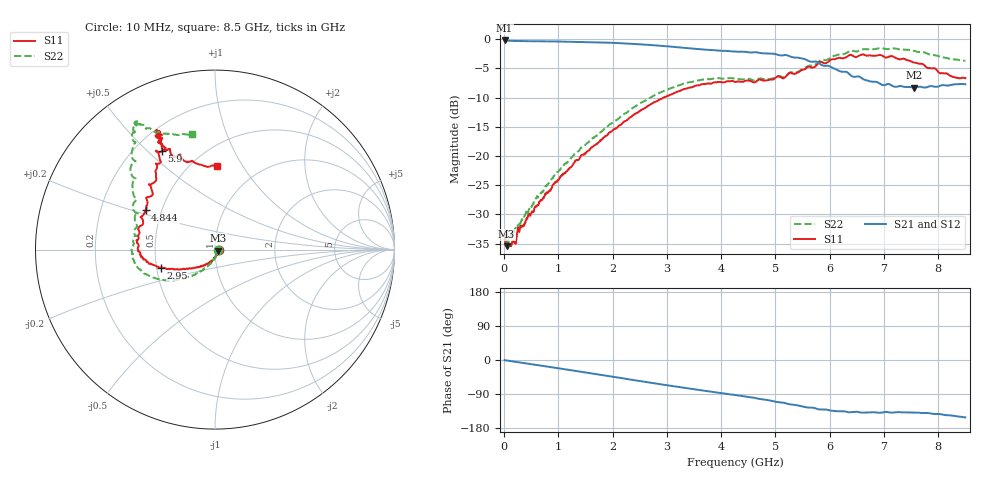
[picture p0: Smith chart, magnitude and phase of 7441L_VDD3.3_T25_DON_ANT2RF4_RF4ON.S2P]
!Agilent Technologies,E5071C,MY46417908,A.11.23
!Date: Mon May 03 19:54:53 2021
!Data & Calibration Information:
!Freq	S11:SOLT2(ON)	S21:SOLT2(ON)	S12:SOLT2(ON)	S22:SOLT2(ON)
!PortZ  Port1:50+j0  Port2:50+j0
!Above PortZ is port z conversion or system Z0 setting when saving the data.
!When reading, reference impedance value at option line is always used.
# Hz S dB R 50
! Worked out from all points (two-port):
!   1601 points, 10 MHz to 8.5 GHz, reference 50 ohm
!   highest |S21| = -0.21 dB at 10 MHz (marker M1); lowest = -8.3 dB at 7.561 GHz (marker M2)
!   |S21| within 3 dB of the highest: start of sweep to 5.456 GHz
!   lowest |S11| = -35.4 dB at 47.14 MHz (marker M3), VSWR 1.03, Z = 51.6 - j0.519 ohm
!   |S11| at or under -10 dB: start of sweep to 2.94 GHz
!   |S22| runs from -34.9 to -1.5 dB; largest |S21 - S12| = 0.0029
!   S11 on the Smith chart (normalised r, x): 10 MHz: 1.04, +0.00; 2.95 GHz: 0.53, -0.12; 4.844 GHz: 0.41, +0.22; 5.9 GHz: 0.31, +0.55; 8.5 GHz: 0.66, +0.78
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1e7  -33.42 0.3  -0.21 -0.4  -0.21 -0.4  -34.47 -9.6
4.714375e7  -35.45 -17.3  -0.26 -1.2  -0.26 -1.2  -34.52 -18.7
1.798e8  -34.69 -40.8  -0.30 -4.1  -0.30 -4.1  -32.84 -45.0
2.806188e8  -33.02 -54.3  -0.30 -6.3  -0.31 -6.3  -31.41 -59.0
4.504188e8  -30.13 -72.0  -0.33 -10.0  -0.33 -10.0  -29.35 -76.4
9.492062e8  -24.55 -101.9  -0.39 -20.7  -0.39 -20.7  -23.28 -103.8
1.426769e9  -19.87 -121.8  -0.47 -31.2  -0.47 -31.2  -18.54 -118.0
2.159031e9  -14.65 -144.9  -0.68 -47.7  -0.68 -47.7  -13.24 -135.1
2.843538e9  -10.45 -160.1  -1.10 -63.3  -1.11 -63.3  -9.27 -150.7
2.949662e9  -9.93 -161.7  -1.18 -65.6  -1.18 -65.6  -8.83 -153.2
3.655394e9  -7.69 -174.2  -1.75 -80.4  -1.74 -80.4  -6.92 -169.2
4.255e9  -7.31 172.2  -2.10 -92.4  -2.10 -92.4  -6.77 177.9
4.843994e9  -7.05 150.4  -2.43 -105.5  -2.42 -105.5  -6.88 163.5
5.204819e9  -6.26 136.5  -2.73 -114.9  -2.71 -115.0  -6.19 155.0
5.671769e9  -4.87 122.8  -3.87 -125.7  -3.84 -125.7  -4.52 138.3
5.899938e9  -4.10 118.5  -4.56 -130.7  -4.54 -130.5  -3.57 132.1
6.372194e9  -2.67 115.8  -6.07 -138.0  -6.10 -137.9  -2.04 125.8
6.658731e9  -2.75 116.3  -7.01 -138.6  -7.00 -138.4  -1.71 122.8
7.088538e9  -3.00 117.1  -7.66 -138.0  -7.67 -138.0  -1.67 122.0
7.560794e9  -4.02 116.0  -8.27 -138.5  -8.29 -138.4  -2.00 119.7
7.932231e9  -4.98 109.9  -8.13 -142.4  -8.17 -142.5  -2.74 116.5
8.5e9  -6.66 88.5  -7.72 -151.5  -7.73 -151.6  -3.65 101.0
